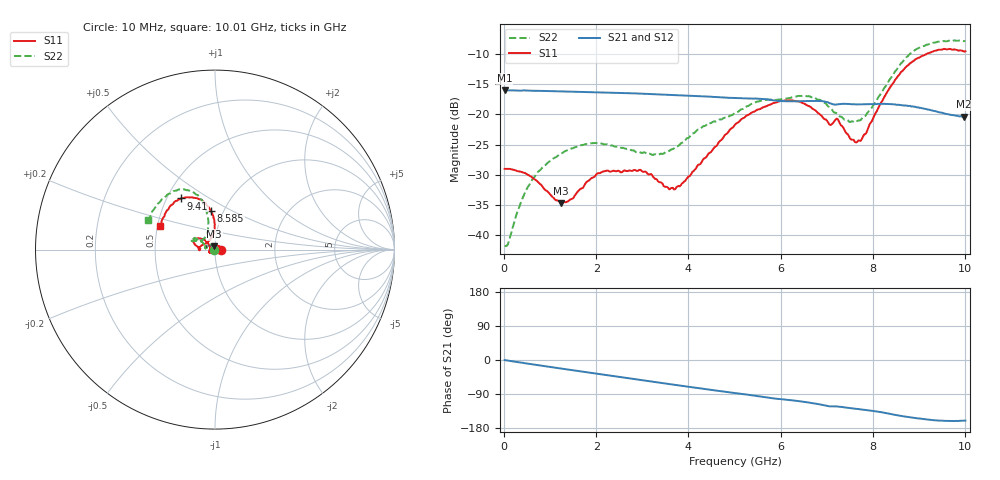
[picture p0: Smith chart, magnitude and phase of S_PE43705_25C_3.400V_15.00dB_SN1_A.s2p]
! Device ID: PE43705
! Serial: 1
! Insertion: A
! Impedance: 50 ohm
! Temp: 25C
! VDD: 3.400V
! Attenuation Step: 15.00dB
#  Hz  S  RI  R  50
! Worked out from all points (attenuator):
!   401 points, 10 MHz to 10.01 GHz, reference 50 ohm
!   highest |S21| = -15.98 dB at 10 MHz (marker M1); lowest = -20.4 dB at 9.985 GHz (marker M2)
!   lowest |S11| = -34.6 dB at 1.235 GHz (marker M3), VSWR 1.04, Z = 49.5 + j1.76 ohm
!   |S11| at or under -10 dB: start of sweep to 9.165 GHz
!   |S22| runs from -41.8 to -7.8 dB; largest |S21 - S12| = 0.0013
!   S11 on the Smith chart (normalised r, x): 10 MHz: 1.07, +0.00; 8.585 GHz: 0.87, +0.39; 9.41 GHz: 0.59, +0.38; 10.01 GHz: 0.52, +0.15
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1e7  0.0355 0.000237  0.1588 -0.000699  0.1589 -0.000649  -0.00818 0.0005
8.5e7  0.0353 0.00248  0.1583 -0.00463  0.1583 -0.00456  -0.00753 0.00395
5.6e8  0.0251 0.0181  0.1546 -0.0285  0.1546 -0.0284  -0.0142 0.0226
1.235e9  -0.00517 0.0178  0.1435 -0.0594  0.1435 -0.0592  -0.0384 0.0275
1.685e9  -0.0236 0.00647  0.1326 -0.0779  0.1326 -0.0779  -0.0518 0.0209
2.21e9  -0.0324 -0.0107  0.117 -0.0972  0.117 -0.097  -0.0559 0.0101
2.96e9  -0.0286 -0.0198  0.0896 -0.1186  0.0898 -0.1186  -0.0475 0.0092
3.36e9  -0.0236 -0.0143  0.0738 -0.1265  0.074 -0.1264  -0.045 0.0121
3.635e9  -0.0243 -0.00453  0.0628 -0.1308  0.0628 -0.1308  -0.0485 0.0174
3.835e9  -0.0256 0.00458  0.0543 -0.1332  0.0543 -0.1332  -0.0525 0.0237
5.01e9  -0.061 0.0552  0.00667 -0.1367  0.00698 -0.1368  -0.0884 0.0531
5.985e9  -0.1147 0.0587  -0.0293 -0.126  -0.0287 -0.1258  -0.1183 0.0603
6.685e9  -0.1092 0.0258  -0.0522 -0.1182  -0.0521 -0.1183  -0.1286 0.0506
7.06e9  -0.0823 0.00515  -0.0662 -0.105  -0.066 -0.1054  -0.1031 0.0499
7.235e9  -0.0913 0.0109  -0.0657 -0.102  -0.0653 -0.1024  -0.0888 0.0478
7.685e9  -0.0346 0.0501  -0.077 -0.0937  -0.0773 -0.0937  -0.0549 0.0703
8.36e9  -0.00371 0.1639  -0.0958 -0.0756  -0.0954 -0.0757  -0.0418 0.1884
8.585e9  -0.0231 0.2143  -0.1002 -0.0654  -0.0993 -0.0659  -0.061 0.2483
8.935e9  -0.0743 0.2776  -0.1032 -0.0516  -0.1026 -0.051  -0.1244 0.322
9.41e9  -0.1878 0.2853  -0.0986 -0.0366  -0.0984 -0.0366  -0.2325 0.3256
9.985e9  -0.2999 0.1402  -0.09 -0.0329  -0.0899 -0.0328  -0.3635 0.1767
1.001e10  -0.3066 0.1314  -0.0901 -0.0329  -0.0904 -0.0336  -0.3712 0.1652
